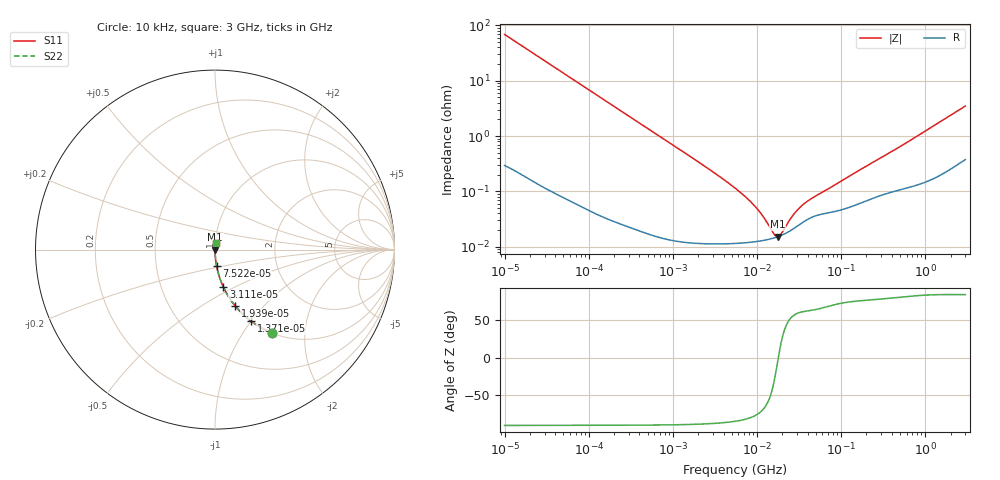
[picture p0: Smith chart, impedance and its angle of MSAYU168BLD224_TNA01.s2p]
! MSAYU168BLD224_TNA01  S-PARAMETER MODEL  ( Standard Model )
! Model Generated by TAIYO YUDEN Corporation (http://www.ty-top.com)
! Version 1.0
! TAIYO YUDEN Control No. 220601
! Copyright(c) 2013 TAIYO YUDEN CO.,LTD. All Rights Reserved.
! Product Description (link to TY-COMPAS)
! https://ds.yuden.co.jp/TYCOMPAS/or/detail?pn=MSAYU168BLD224KTNA01&u=M
! Products Name : Multilayer Ceramic Capacitors
! Characteristics :
!  Capacitance : 0.22 [uF] , Rated Voltage : 50 [V] , TCC : X5R
!  Case Size : 1.6 x 0.8 / 0.063 x 0.031 [mm/inch] , Thickness : 0.8 / 0.031 [mm/inch]
!  (Conditions: Temperature = 25 [degC] , DC Bias Voltage = 0 [V])
! External Node Assignments :
!  1  o---| |---o  2
! GND o---------o GND
! Frequency Range : 10kHz  -  3GHz  [ 401 STEP ]
# MHZ S RI R 50
! Freq[MHz].  S11 Real  S11 Imag  S21 Real  S21 Imag  S12 Real  S12 Imag  S22 Real  S22 Imag
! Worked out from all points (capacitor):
!   401 points, 10 kHz to 3 GHz, reference 50 ohm
!   read as one part in series: C = 233 nF near 10.65 kHz
!   lowest |Z| = 15.2 mohm at 17.59 MHz (marker M1)
!   series resonance near 17.92 MHz, so ESL is about 340 pH
!   S11 on the Smith chart (normalised r, x): 10 kHz: 1.01, -1.37; 13.71 kHz: 1.00, -1.00; 19.39 kHz: 1.00, -0.71; 31.11 kHz: 1.00, -0.44; 75.22 kHz: 1.00, -0.18; 3 GHz: 1.01, +0.07
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0.01  0.3186 -0.4638  0.6814 0.4638  0.6814 0.4638  0.3186 -0.4638
0.013707  0.2002 -0.3978  0.7998 0.3978  0.7998 0.3978  0.2002 -0.3978
0.019389  0.1119 -0.3128  0.8881 0.3128  0.8881 0.3128  0.1119 -0.3128
0.031113  0.0472 -0.2095  0.9528 0.2095  0.9528 0.2095  0.0472 -0.2095
0.075221  0.00882 -0.0905  0.9912 0.0905  0.9912 0.0905  0.00882 -0.0905
0.082683  0.00737 -0.0824  0.9926 0.0824  0.9926 0.0824  0.00737 -0.0824
0.199902  0.00147 -0.0344  0.9985 0.0344  0.9985 0.0344  0.00147 -0.0344
0.683653  0.00025 -0.0101  0.9998 0.0101  0.9998 0.0101  0.00025 -0.0101
2.652321  0.000119 -0.00256  0.9999 0.00256  0.9999 0.00256  0.000119 -0.00256
5.477226  0.000116 -0.00114  0.9999 0.00114  0.9999 0.00114  0.000116 -0.00114
7.507384  0.000119 -0.000758  0.9999 0.000758  0.9999 0.000758  0.000119 -0.000758
9.6612  0.000124 -0.000506  0.9999 0.000506  0.9999 0.000506  0.000124 -0.000506
12.04705  0.000131 -0.000313  0.9999 0.000313  0.9999 0.000313  0.000131 -0.000313
15.99985  0.000145 -8.67e-05  0.9999 8.67e-05  0.9999 8.67e-05  0.000145 -8.67e-05
17.5871  0.000151 -1.42e-05  0.9998 1.42e-05  0.9998 1.42e-05  0.000151 -1.42e-05
19.33182  0.00016 5.79e-05  0.9998 -5.79e-05  0.9998 -5.79e-05  0.00016 5.79e-05
24.87798  0.000195 0.000249  0.9998 -0.000249  0.9998 -0.000249  0.000195 0.000249
30.05882  0.000235 0.000391  0.9998 -0.000391  0.9998 -0.000391  0.000235 0.000391
36.31858  0.000286 0.000526  0.9997 -0.000526  0.9997 -0.000526  0.000286 0.000526
45.28751  0.000344 0.000675  0.9997 -0.000675  0.9997 -0.000675  0.000344 0.000675
374.4521  0.000967 0.00486  0.999 -0.00486  0.999 -0.00486  0.000967 0.00486
3000  0.00492 0.0344  0.9951 -0.0344  0.9951 -0.0344  0.00492 0.0344
